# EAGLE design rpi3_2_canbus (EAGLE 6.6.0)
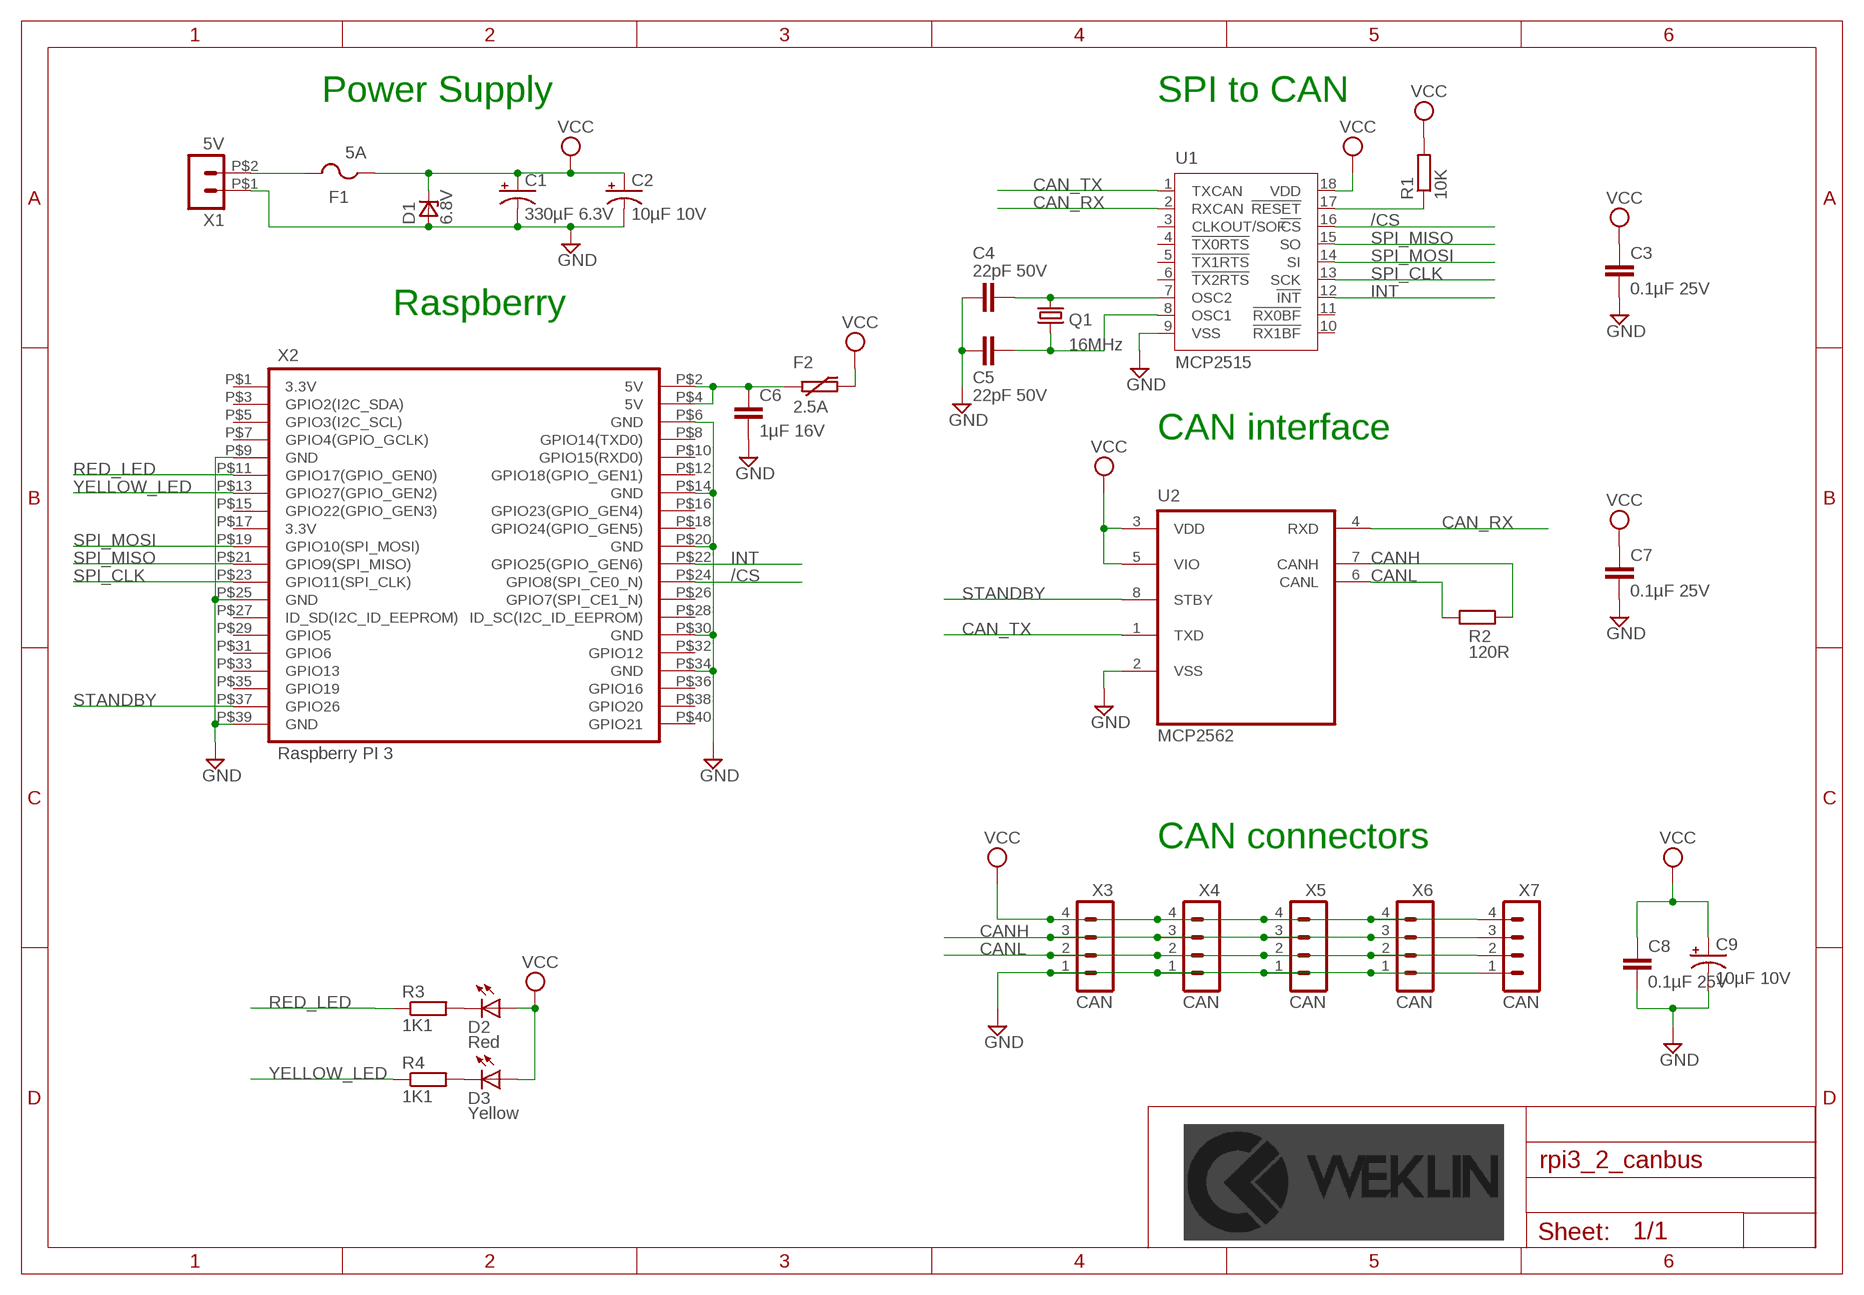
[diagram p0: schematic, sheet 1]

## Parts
C1  330µF 6.3V  CAPACITOR_POL-330µF-6.3V(+-10%)(7343)  [EIA7343]
C2  10µF 10V  CAPACITOR_POL-10µF-10V(+-10%)(3216)  [EIA3216]
C3  0.1µF 25V  CAPACITOR_NON_POL-100NF-25V(+-10%)(2012)  [C2012]
C4  22pF 50V  CAPACITOR_NON_POL-22PF-50V(+-5%)(2012)  [C2012]
C5  22pF 50V  CAPACITOR_NON_POL-22PF-50V(+-5%)(2012)  [C2012]
C6  1µF 16V  CAPACITOR_NON_POL-1µF-16V(-20%)(2012)  [C2012]
C7  0.1µF 25V  CAPACITOR_NON_POL-100NF-25V(+-10%)(2012)  [C2012]
C8  0.1µF 25V  CAPACITOR_NON_POL-100NF-25V(+-10%)(2012)  [C2012]
C9  10µF 10V  CAPACITOR_POL-10µF-10V(+-10%)(3216)  [EIA3216]
D1  6.8V  ZENER_UNIDIR6.8  [DO-214AA]
D2  Red  LEDVLDS1235G  [VLD]
D3  Yellow  LED-VLDY1235G  [VLD]
F1  5A  FUSE04510451005.NRL  [EIARS-481-2]
F2  2.5A  PTCFUSE-2.5A-4532(1812)  [F4532]
Q1  16MHz  CRYSTAL-16MHZ_SMD(3225)  [SMD_KX7]
R1  10K  RESISTOR-10K(+-1%)(2012)  [R2012]
R2  120R  RESISTOR-120R(+-1%)(2012)  [R2012]
R3  1K1  RESISTOR-1K1(+-1%)(2012)  [R2012]
R4  1K1  RESISTOR-1K1(+-1%)(2012)  [R2012]
U1  MCP2515  MCP2515SOIC18  [SOIC18]
U2  MCP2562  MCP2562-E/SN-SOIC8  [SOIC8]
X1  5V  HEADER_POS2_43650-0212  [43650-0212]
X2  Raspberry PI 3  RPI3  [RPI3]
X3  CAN  MICROLOCK-4CMS_HORIZONTAL  [504195-0470]
X4  CAN  MICROLOCK-4CMS_HORIZONTAL  [504195-0470]
X5  CAN  MICROLOCK-4CMS_HORIZONTAL  [504195-0470]
X6  CAN  MICROLOCK-4CMS_HORIZONTAL  [504195-0470]
X7  CAN  MICROLOCK-4CMS_HORIZONTAL  [504195-0470]

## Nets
/CS: U1.16(!CS) X2.P$24(GPIO8(SPI_CE0_N))
CAN_RX: U1.2(RXCAN) U2.4(RXD)
CAN_TX: U1.1(TXCAN) U2.1(TXD)
CANH: R2.1 U2.7(CANH) X3.3 X4.3 X5.3 X6.3 X7.3
CANL: R2.2 U2.6(CANL) X3.2 X4.2 X5.2 X6.2 X7.2
GND: C1.C(-) C2.C(-) C3.2 C4.1 C5.1 C6.2 C7.2 C8.2 C9.C(-) D1.A U1.9(VSS) U2.2(VSS) X1.P$1 X2.P$6(GND) X2.P$9(GND) X2.P$14(GND) X2.P$20(GND) X2.P$25(GND) X2.P$30(GND) X2.P$34(GND) X2.P$39(GND) X3.1 X4.1 X5.1 X6.1 X7.1
INT: U1.12(!INT) X2.P$22(GPIO25(GPIO_GEN6))
N$1: F1.2 X1.P$2
N$3: R1.1 U1.17(!RESET)
N$4: C4.2 Q1.3 U1.7(OSC2)
N$5: C6.1 F2.1 X2.P$2(5V) X2.P$4(5V)
N$7: C5.2 Q1.1 U1.8(OSC1)
N$8: D3.C R4.2
N$9: D2.C R3.2
RED_LED: R3.1 X2.P$11(GPIO17(GPIO_GEN0))
SPI_CLK: U1.13(SCK) X2.P$23(GPIO11(SPI_CLK))
SPI_MISO: U1.15(SO) X2.P$21(GPIO9(SPI_MISO))
SPI_MOSI: U1.14(SI) X2.P$19(GPIO10(SPI_MOSI))
STANDBY: U2.8(STBY) X2.P$37(GPIO26)
VCC: C1.A(+) C2.A(+) C3.1 C7.1 C8.1 C9.A(+) D1.C D2.A D3.A F1.1 F2.2 R1.2 U1.18(VDD) U2.3(VDD) U2.5(VIO) X3.4 X4.4 X5.4 X6.4 X7.4
YELLOW_LED: R4.1 X2.P$13(GPIO27(GPIO_GEN2))
Unconnected: U1.3(CLKOUT/SOF) U1.4(!TX0RTS) U1.5(!TX1RTS) U1.6(!TX2RTS) U1.10(!RX1BF) U1.11(!RX0BF) X2.P$1(3.3V) X2.P$3(GPIO2(I2C_SDA)) X2.P$5(GPIO3(I2C_SCL)) X2.P$7(GPIO4(GPIO_GCLK)) X2.P$8(GPIO14(TXD0)) X2.P$10(GPIO15(RXD0)) X2.P$12(GPIO18(GPIO_GEN1)) X2.P$15(GPIO22(GPIO_GEN3)) X2.P$16(GPIO23(GPIO_GEN4)) X2.P$17(3.3V) X2.P$18(GPIO24(GPIO_GEN5)) X2.P$26(GPIO7(SPI_CE1_N)) X2.P$27(ID_SD(I2C_ID_EEPROM)) X2.P$28(ID_SC(I2C_ID_EEPROM)) X2.P$29(GPIO5) X2.P$31(GPIO6) X2.P$32(GPIO12) X2.P$33(GPIO13) X2.P$35(GPIO19) X2.P$36(GPIO16) X2.P$38(GPIO20) X2.P$40(GPIO21)

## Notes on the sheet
- Power Supply | SPI to CAN
- Raspberry
- CAN interface
- CAN connectors

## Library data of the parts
C1 = weklin_capacitor:CAPACITOR_POL: Capacitor; LIB: weklin_capacitor; MANUFACTURER: Kemet; MPN: T491D337K006AT; OC_FARNELL: 2313928; PRICE: 0,497
C2 C9 = weklin_capacitor:CAPACITOR_POL: Capacitor; LIB: weklin_capacitor; MANUFACTURER: Kemet; MPN: T491A106K010AT; OC_FARNELL: 2250086; PRICE: 0,0578
C3 C7 C8 = weklin_capacitor:CAPACITOR_NON_POL: Condensateur céramique multicouche; LIB: weklin_capacitor; MANUFACTURER: AVX; MPN: 08053C104KAT2A; OC_FARNELL: 2280951; PRICE: 0,0036
C4 C5 = weklin_capacitor:CAPACITOR_NON_POL: Condensateur céramique multicouche; LIB: weklin_capacitor; MANUFACTURER: Multicomp; MPN: MC0805N220J500CT; OC_FARNELL: 2310684; PRICE: 0,0078
C6 = weklin_capacitor:CAPACITOR_NON_POL: Condensateur céramique multicouche; LIB: weklin_capacitor; MANUFACTURER: Walsin; MPN: 0805F105Z160CT; OC_FARNELL: 2495495; PRICE: 0,0097
D1 = weklin_diode:ZENER_UNIDIR: P6SMBxxA Series of unidirectional Transient Voltage Suppressor Diodes; LIB: weklin_diode; MANUFACTURER: ON Semiconductor; MPN: P6SMB6.8AT3G; OC_FARNELL: 1459166RL; PRICE: 0,178
D2 = weklin_led:LED: Led; LIB: weklin_led; MANUFACTURER: Vishay; MPN: VLDS1235G; OC_FARNELL: 2494682; PRICE: 0,003
D3 = weklin_led:LED: Led; LIB: weklin_led; MANUFACTURER: Vishay; MPN: VLDY1235G; OC_FARNELL: 2494684; PRICE: 0,003
F1 = weklin_fuse:FUSE: Fuse; LIB: weklin_fuse; MANUFACTURER: Littlefuse; MPN: 0451005.NRL; OC_FARNELL: 9922199; PRICE: 2,02
F2 = weklin_fuse:PTCFUSE: Fuse time lag; LIB: weklin_fuse; MANUFACTURER: Bourns; MPN: MF-MSMF250/16X-2; OC_FARNELL: 2250006; PRICE: 0,82
Q1 = weklin_crystal:CRYSTAL: Crystal resonator; LIB: weklin_crystal; MANUFACTURER: AEL CRYSTALS; MPN: E3SB16.0000F09G11AE; OC_FARNELL: 2467444RL; PRICE: 0,315
R1 = weklin_resistor:RESISTOR: Resistor; LIB: weklin_resistor; MANUFACTURER: Multicomp; MPN: MCWR08X1002FTL; OC_FARNELL: 2446870; PRICE: 0,0014
R2 = weklin_resistor:RESISTOR: Resistor; LIB: weklin_resistor; MANUFACTURER: Multicomp; MPN: MCWR08X1200FTL; OC_FARNELL: 2446878; PRICE: 0,0014
R3 R4 = weklin_resistor:RESISTOR: Resistor; LIB: weklin_resistor; MANUFACTURER: Multicomp; MPN: MC0805S8F1101T5E; OC_FARNELL: 1635316; PRICE: 0,003
U1 = weklin_ic_can:MCP2515: Stand-Alone CAN Controller With SPI Interface; LIB: weklin_ic_can; MANUFACTURER: Microchip; MPN: MCP2515-I/SO; OC_FARNELL: 1292239; PRICE: 1,9
U2 = weklin_ic_can:MCP2562-E/SN: High-Speed CAN Transceiver; LIB: weklin_ic_can; MANUFACTURER: Microchip; MPN: MCP2562-E/SN; OC_FARNELL: 2362839; PRICE: 1,12
X1 = weklin_micro_fit:HEADER_POS2_?: Molex - Micro-Fit 3.0 Series connector, 2 way; LIB: weklin_micro_fit; MANUFACTURER: Molex; MPN: 43650-0213; OC_FARNELL: 2396411; PRICE: 1,12
X2 = weklin_raspberry:RPI3: Raspberry PI3 Model B; LIB: weklin_raspberry; MANUFACTURER: Harwin; MPN: M20-6102045; OC_FARNELL: 1569230; PRICE: 4,24
X3-X7 = weklin_micro-lock:MICROLOCK-4: Connecteur MOLEX de 4 Contacts Série Mini50 GEII/IUT ANGERS; LIB: weklin_micro-lock; MANUFACTURER: Molex; MPN: 504195-0470; OC_FARNELL: 2445490; PRICE: 0,713

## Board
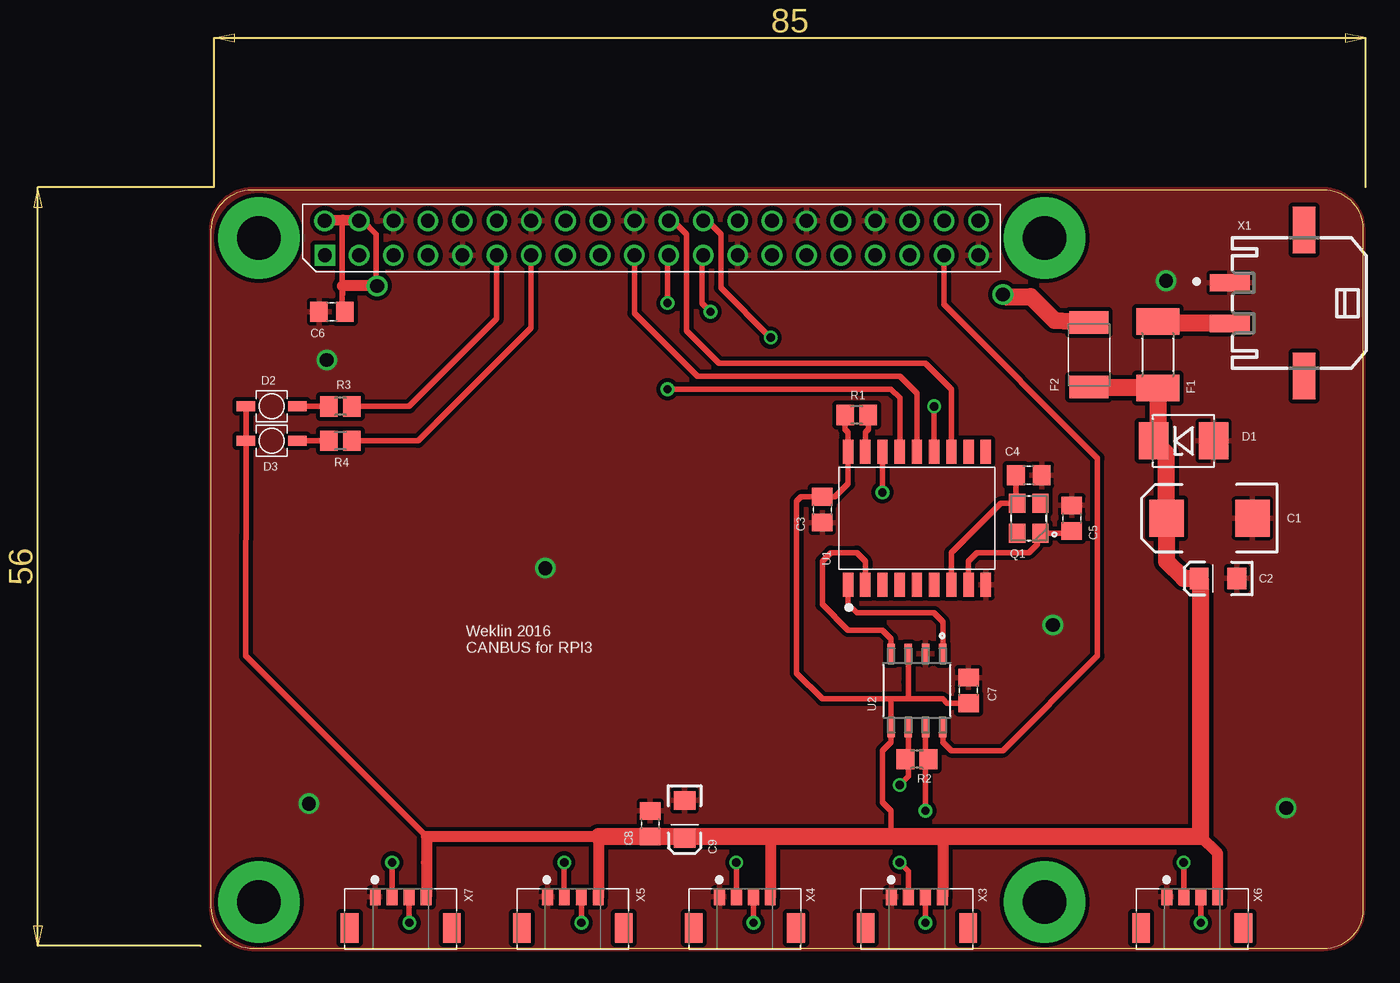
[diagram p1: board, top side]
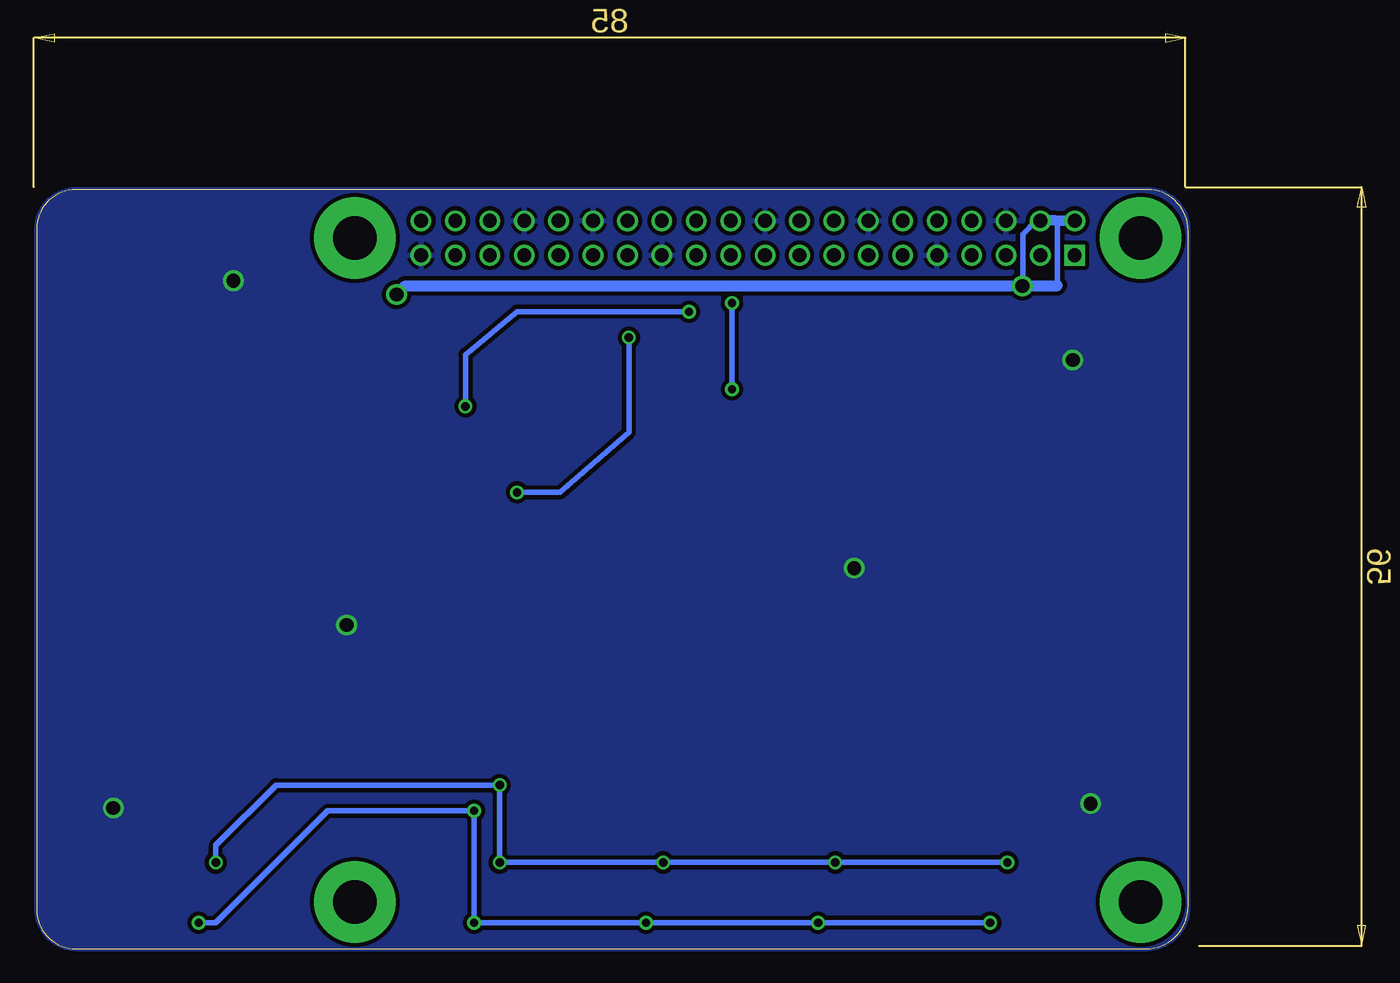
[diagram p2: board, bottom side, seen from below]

Size 98.3 x 67.5 mm. Coordinates in mm from the lower left corner, seen from the top.
Outline: 13.1,3.1 13.1,53 arc-90 16.1,56 95.2,56 arc-90 98.1,53.1 98.1,2.9 arc-90 95.2,0 16.2,0 arc-90 13.1,3.1
Copper layers (1*16): Top 0.035mm / dielectric 1.5mm / Bottom 0.035mm
Design rules "default *": minimum track width 10mil, minimum drill 24mil, track to track 12mil, track to pad 10mil, pad to pad 8mil, via to via 8mil, smd to smd 8mil, copper to edge 0mil, drill to drill 8mil, minimum pad ring 10mil, minimum via ring 8mil, stop-mask expansion 4mil, vias tented up to drill 0mil, thermal gap 10mil

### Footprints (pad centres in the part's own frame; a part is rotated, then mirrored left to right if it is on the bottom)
EIA7343 = smd 2.55 x 2.7: A 3.17,0; C -3.17,0
EIA3216 = smd 1.4 x 1.6: A 1.4,0; C -1.4,0
C2012 = smd 1.3 x 1.5: 1 -0.95,0; 2 0.95,0
DO-214AA = smd 2.159 x 2.743: A 2.21,0; C -2.21,0
VLD = smd 1.35 x 0.75: A 1.9,0; C -1.9,0
EIARS-481-2 = smd 1.956 x 3.15: 1 -2.451,0; 2 2.451,0
F4532 = smd 1.676 x 2.896: 1 -2.388,0; 2 2.388,0
SMD_KX7 = smd 1.4 x 1.2: 1 -1.1,-0.85; 2 1.1,-0.85; 3 1.1,0.85; 4 -1.1,0.85
R2012 = smd 1.3 x 1.5: 1 -0.85,0; 2 0.85,0
SOIC18 = smd 0.762 x 1.778: 1 -5.08,-4.915; 2 -3.81,-4.915; 3 -2.54,-4.915; 4 -1.27,-4.915; 5 0,-4.915; 6 1.27,-4.915; 7 2.54,-4.915; 8 3.81,-4.915; 9 5.08,-4.915; 10 5.08,4.915; 11 3.81,4.915; 12 2.54,4.915; 13 1.27,4.915; 14 0,4.915; 15 -1.27,4.915; 16 -2.54,4.915; 17 -3.81,4.915; 18 -5.08,4.915
SOIC8 = smd 1.473 x 0.559: 1 -2.718,1.905; 2 -2.718,0.635; 3 -2.718,-0.635; 4 -2.718,-1.905; 5 2.718,-1.905; 6 2.718,-0.635; 7 2.718,0.635; 8 2.718,1.905
43650-0212 = smd 2.92 x 1.27: P$1 -5.48,1.5; P$2 -5.48,-1.5 | smd 1.65 x 3.43: TAB1 0,5.38; TAB2 0,-5.38
RPI3 = drill 3.2 pad 6: 1 -28.987,-0.002; 2 29.013,-49.002; 3 29.013,-0.002; 4 -28.987,-49.002 | drill 1.016 square: P$1 -24.117,-1.272 | drill 1.016: P$2 -24.13,1.27; P$3 -21.59,-1.27; P$4 -21.59,1.27; P$5 -19.05,-1.27; P$6 -19.05,1.27; P$7 -16.51,-1.27; P$8 -16.51,1.27; P$9 -13.97,-1.27; P$10 -13.97,1.27; P$11 -11.43,-1.27; P$12 -11.43,1.27; P$13 -8.89,-1.27; P$14 -8.89,1.27; P$15 -6.35,-1.27; P$16 -6.35,1.27; P$17 -3.81,-1.27; P$18 -3.81,1.27; P$19 -1.27,-1.27; P$20 -1.27,1.27; P$21 1.27,-1.27; P$22 1.27,1.27; P$23 3.81,-1.27; P$24 3.81,1.27; P$25 6.35,-1.27; P$26 6.35,1.27; P$27 8.89,-1.27; P$28 8.89,1.27; P$29 11.43,-1.27; P$30 11.43,1.27; P$31 13.97,-1.27; P$32 13.97,1.27; P$33 16.51,-1.27; P$34 16.51,1.27; P$35 19.05,-1.27; P$36 19.05,1.27; P$37 21.59,-1.27; P$38 21.59,1.27; P$39 24.13,-1.27; P$40 24.13,1.27
504195-0470 = smd 0.8 x 1.2: 1 1.875,0; 2 0.625,0; 3 -0.625,0; 4 -1.875,0 | smd 1.3 x 2.15: P$5 -3.775,2.295; P$6 3.775,2.295

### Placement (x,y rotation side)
C1  86.77,31.76 180 top
C2  87.41,27.31 180 top
C3  58.2,32.4 270 top
C4  73.44,34.94 180 top
C5  76.61,31.76 270 top
C6  22,47 180 top
C7  68.99,19.06 90 top
C8  45.5,9.22 90 top
C9  48.03,9.54 270 top
D1  84.86,37.48 0 top
D2  17.55,40.02 180 top
D3  17.55,37.48 180 top
DRILEGEND  [DRILEGEND]  not placed on the board
F1  82.96,43.83 90 top
F2  77.88,43.83 270 top
Q1  73.44,31.76 90 top
R1  60.73,39.38 180 top
R2  65.18,13.98 180 top
R3  22.64,40.02 180 top
R4  22.64,37.48 180 top
U1  65.18,31.76 0 top
U2  65.18,19.06 270 top
X1  93.75,47.64 0 top
X2  45.6,52.44 0 top
X3  65.18,3.82 180 top
X4  52.48,3.82 180 top
X5  39.78,3.82 180 top
X6  85.5,3.82 180 top
X7  27.08,3.82 180 top

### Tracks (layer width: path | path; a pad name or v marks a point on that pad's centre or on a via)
/CS  (via drill 0.61)
  Top 0.406: X2.P$24 49.64,53.78 50.7,52.72 50.7,48.78 v54.39,45.1 | U1.16 v62.64,33.67
  Bottom 0.406: v62.64,33.67 59.47,33.67 54.39,38.11 v54.39,45.1
CAN_RX
  Top 0.406: U2.4 63.28,22.87 62.64,23.5 60.1,23.5 58.2,25.41 58.2,28.58 58.83,29.22 60.73,29.22 61.37,28.58 U1.2
CAN_TX
  Top 0.406: U1.1 60.1,25.41 60.73,24.77 66.45,24.77 67.08,24.14 U2.1
CANH  (via drill 0.61)
  Top 0.406: X7.3 27.71,1.92 v27.71,1.92 | v40.41,1.92 X5.3 | X4.3 53.11,1.92 v53.11,1.92 | X3.3 65.81,1.92 v65.81,1.92 | U2.7 65.81,13.98 | 65.81,13.98 v65.81,10.17 | X6.3 86.12,1.92 v86.13,1.92 | R2.1 65.81,13.98
  Bottom 0.406: v27.71,1.92 v40.41,1.92 v53.11,1.92 v65.81,1.92 v65.81,10.17 75.97,10.17 76.61,10.17 84.86,1.92 v86.13,1.92
CANL  (via drill 0.61)
  Top 0.406: X7.2 26.46,6.35 v26.45,6.36 | v39.14,6.36 39.14,3.83 X5.2 | X4.2 v51.86,6.35 v51.84,6.36 | X3.2 64.56,5.72 v63.91,6.36 | X6.2 84.88,6.35 v84.86,6.36 | v63.91,12.07 64.55,12.71 64.55,13.98 | 64.55,13.98 U2.6 | R2.2 64.55,13.98
  Bottom 0.406: v26.45,6.36 v39.14,6.36 v51.84,6.36 v63.91,6.36 v63.91,12.07 80.42,12.07 84.86,7.63 v84.86,6.36
GND  (via drill 1.02)
  other vias: 75.21,23.89 37.75,28.08 20.3,10.7 92.43,10.37 83.57,49.29 21.62,43.44
  pour Bottom: 13.11,52.97 arc-90 16.16,56.02 95.15,56.02 arc-90 98.07,53.1 98.07,2.93 arc-90 95.15,0.01 16.16,0.01 arc-90 13.11,3.19
  pour Top: 13.11,52.97 arc-90 16.16,56.02 95.15,56.02 arc-90 98.07,53.1 98.07,2.93 arc-90 95.15,0.01 16.16,0.01 arc-90 13.11,3.19
INT
  Top 0.406: X2.P$22 47.09,53.78 48.16,52.72 48.16,45.6 50.58,43.19 65.81,43.19 67.72,41.29 U1.12
N$1
  Top 0.813: 83.1,46.14 F1.2
  Top 1.27: X1.P$2 83.1,46.14
N$3
  Top 0.406: U1.17 61.37,38.11 61.58,38.33 R1.1
N$4
  Top 0.406: U1.7 67.72,29.22 71.36,32.86 Q1.3 72.48,32.96 C4.2
N$5  (via drill 1.02)
  Top 0.406: 25.27,49 25.27,52.72 24.23,53.78 X2.P$4 | 22.77,47.48 22.79,48.91 v25.33,48.91 | 22.77,47.48 22.79,47.16 C6.1 | 22.76,48.91 22.76,52.24 | 22.76,53.83 22.81,53.78 | 22.76,53.83 22.72,53.78 X2.P$2 | 22.76,53.83 22.77,53.79 22.77,47.48 | 22.76,53.83 22.76,49.38
  Top 0.813: 71.68,48.12 v71.53,48.27 | X2.P$2 22.81,53.78 X2.P$4 24.08,53.78 arc90 24.1,53.8 | 25.27,49 25.2,48.91 22.79,48.91 22.76,48.91
  Top 1.27: 71.68,48.12 73.59,48.12 75.34,46.37 F2.1
  Bottom 0.406: X2.P$2 21.7,53.78 | 22.76,53.83 22.76,48.94 | 25.3,49.25 25.3,52.72 24.27,53.78
  Bottom 0.813: v71.53,48.27 70.89,48.91 v25.33,48.91 22.79,48.91 22.76,48.94 | 24.27,53.78 X2.P$2
N$7
  Top 0.406: U1.8 68.99,28.58 69.62,29.22 73.44,29.22 74.07,29.86 74.07,30.44 Q1.1 76.46,30.66 C5.2
N$8
  Top 0.406: D3.C R4.2
N$9
  Top 0.406: D2.C R3.2
RED_LED
  Top 0.406: R3.1 27.71,40.02 34.17,46.47 X2.P$11
SPI_CLK  (via drill 0.61)
  Top 0.406: U1.13 v66.45,40.02 | v49.94,47 49.31,47.64 49.31,51.14 X2.P$23
  Bottom 0.406: v66.45,40.02 66.45,43.83 62.64,47 v49.94,47
SPI_MISO  (via drill 0.61)
  Top 0.406: U1.15 63.91,40.65 63.28,41.29 v46.77,41.29 | v46.77,47.64 46.77,51.14 X2.P$21
  Bottom 0.406: v46.77,41.29 v46.77,47.64
SPI_MOSI
  Top 0.406: X2.P$19 44.33,46.9 48.99,42.24 63.91,42.24 65.18,40.97 U1.14
STANDBY
  Top 0.406: U2.8 67.08,15.25 67.72,14.61 71.53,14.61 78.52,21.6 78.52,36.21 67.19,47.53 X2.P$37
VCC
  Top 0.406: R1.2 59.89,38.33 60.1,38.11 U1.18 60.1,34.3 59.14,33.35 | C3.1 59.14,33.35 | U2.3 64.55,19.7 64.55,18.43 | 63.28,8.27 63.28,10.17 62.64,10.8 62.64,14.61 63.28,15.25 U2.5 63.28,18.43 62.64,18.43 | 59.14,33.35 56.61,33.35 56.29,33.03 56.29,20.33 58.2,18.43 62.64,18.43 | C7.1 67.4,18.11 67.08,18.43 64.55,18.43 | 64.55,18.43 62.64,18.43 | D2.A D3.A 15.66,30.48 15.65,29.86 15.65,21.6 28.98,8.27
  Top 0.813: X6.4 87.38,7.02 86.13,8.27 | 67.08,8.27 67.08,3.85 X3.4 | 54.39,8.27 54.39,3.85 X4.4 | X5.4 41.69,3.85 41.69,8.27 28.98,8.27 28.98,6.36 28.98,3.85 X7.4 | C9.A 48.03,8.27 | C8.1 46.13,8.27 | 82.96,37.78 D1.C | 86.13,27.18 C2.A
  Top 1.27: 41.69,8.27 46.13,8.27 48.03,8.27 54.39,8.27 63.28,8.27 67.08,8.27 86.13,8.27 86.13,27.18 | 82.96,37.78 F1.1 78.58,41.37 78.52,41.44 F2.2 | D1.C 83.6,36.53 C1.A 83.6,28.58 84.86,27.31 C2.A
YELLOW_LED
  Top 0.406: X2.P$13 36.71,45.83 28.35,37.48 R4.1

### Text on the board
tPlace: Weklin 2016 / CANBUS for RPI3
DrillLegend: LAYER-STACK
DrillLegend_01-16: 01-16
